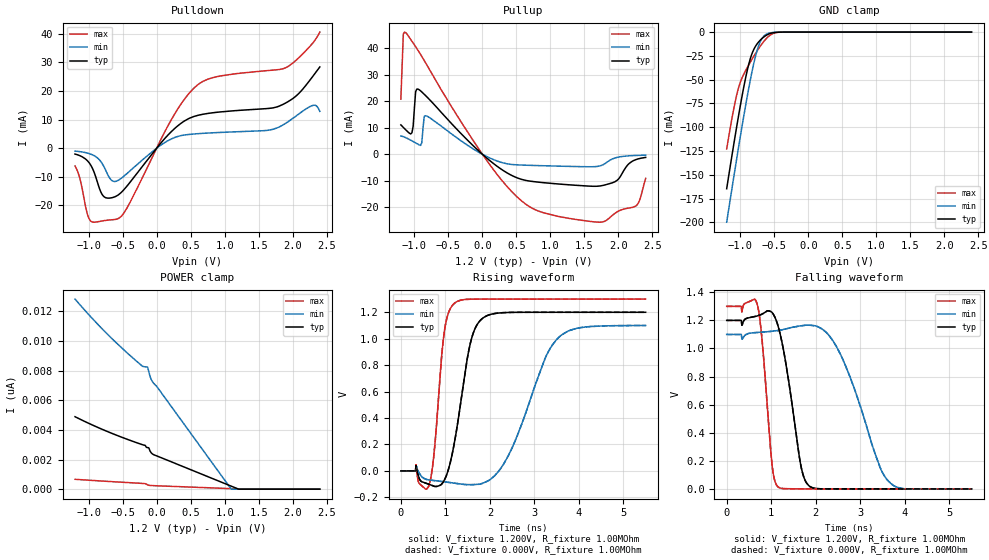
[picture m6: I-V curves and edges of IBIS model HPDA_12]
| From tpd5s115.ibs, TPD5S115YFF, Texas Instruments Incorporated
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[Model]   HPDA_12
Model_type   I/O
Vinl = 0.4V
Vinh = 1.0V
Vmeas = 1.500V
Vref = 0V
Cref =15pF
|   typ   min   max
|3-state
C_comp   1.5724pF   1.4611pF   1.8386pF
|pulldown
|C_comp   1.6216pF   1.4827pF   1.9515pF
|pullup
|C_comp   1.689pF   1.5267pF   2.0704pF
[Voltage Range]   1.200V   1.10V   1.30V
|Junction temperature
[Temperature Range]   40.0   100.0   -40.0
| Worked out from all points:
|   slope of the pulldown table from 0 to 0.18 V, typ, clamps not added: 36.5 ohm
|   slope of the pullup table from 0 to 0.18 V, typ, clamps not added: 47.1 ohm
|   GND clamp passes 1 mA (typ) near -0.54 V on its own axis
|   falling waveform, V_fixture 1.200V, R_fixture 1.00MOhm: 20-80 % time 333ps typ, 703ps min, 192ps max; typ from 1.2 V to 0 V
|   rising waveform, V_fixture 1.200V, R_fixture 1.00MOhm: 20-80 % time 340ps typ, 720ps min, 191ps max; typ from 0 V to 1.2 V
|   rising waveform, V_fixture 0.000V, R_fixture 1.00MOhm: 20-80 % time 340ps typ, 720ps min, 191ps max; typ from 0 V to 1.2 V
|   falling waveform, V_fixture 0.000V, R_fixture 1.00MOhm: 20-80 % time 333ps typ, 703ps min, 192ps max; typ from 1.2 V to 0 V
|ambient temperature   25   85   -40|
[Pulldown]
|   Voltage   I(typ)   I(min)   I(max)
-1.2V     -2.038mA   -994.7uA   -6.215mA
-982.9mV  -5.39mA    -1.945mA   -25.1mA
-783.9mV  -16.73mA   -6.042mA   -25.37mA
-675.4mV  -17.39mA   -10.91mA   -25.06mA
-566.8mV  -16.37mA   -11.25mA   -24.61mA
-385.9mV  -11.76mA   -7.802mA   -18.7mA
138.7mV   3.893mA    2.257mA    6.602mA
554.8mV   11.16mA    4.996mA    21.17mA
880.4mV   12.56mA    5.465mA    25mA
1.803V    14.74mA    7.446mA    27.54mA
2.291V    24.98mA    14.93mA    36.66mA
2.4V      28.44mA    12.91mA    40.63mA
[GND Clamp]
|   Voltage   I(typ)   I(min)   I(max)
-1.2V     -164.7mA   -199.9mA   -122.9mA
-1.11V    -124.1mA   -158.6mA   -85.69mA
-1.037V   -92.89mA   -126.4mA   -61.66mA
-982.9mV  -70.79mA   -102.8mA   -49.69mA
-874.4mV  -33.52mA   -58.6mA    -34.37mA
-820.1mV  -21.26mA   -39.03mA   -27.68mA
-747.7mV  -11.93mA   -18.1mA    -19.3mA
-693.5mV  -7.572mA   -8.233mA   -13.56mA
-639.2mV  -4.359mA   -3.305mA   -8.543mA
-530.7mV  -894.9uA   -472.7uA   -1.914mA
-404mV    -67.45uA   -43.38uA   -90.57uA
2.4V      0A         0A         0A
[Pullup]
|   Voltage   I(typ)   I(min)   I(max)
-1.2V     11.11mA    6.899mA    20.81mA
-1.164V   10.16mA    6.66mA     45.34mA
-1.146V   9.692mA    6.482mA    46.11mA
-1.037V   8.113mA    5.089mA    42.66mA
-982.9mV  23.63mA    4.314mA    40.6mA
-946.7mV  24.59mA    3.797mA    39.18mA
-892.5mV  23.54mA    4.317mA    36.94mA
-838.2mV  22.19mA    14.56mA    34.6mA
681.4mV   -10.04mA   -4.14mA    -19.58mA
1.767V    -11.76mA   -4.006mA   -25.49mA
2.273V    -1.845mA   -410.4uA   -19.07mA
2.4V      -1.169mA   -315.3uA   -9.052mA
[POWER Clamp]
|   Voltage   I(typ)   I(min)   I(max)
-1.2V     4.894nA    12.84nA    666.9pA
-874.4mV  4.189nA    11.18nA    569.1pA
-530.7mV  3.538nA    9.615nA    473.7pA
-205mV    2.998nA    8.296nA    384.9pA
-132.7mV  2.807nA    8.242nA    288.7pA
-114.6mV  2.792nA    7.924nA    264.5pA
-96.48mV  2.574nA    7.608nA    253.3pA
-60.3mV   2.374nA    7.251nA    242.1pA
0V        2.251nA    6.951nA    228.7pA
1.097V    202.6pA    0A         35.11pA
1.206V    0A         0A         15.96pA
2.4V      0A         0A         0A
[Ramp]
R_load = 1.00MOhm
|   typ   min   max
dV/dt_r   719.939mV/340.267ps 659.894mV/720.118ps 779.961mV/190.699ps
dV/dt_f   719.946mV/333.102ps 659.906mV/703.346ps 779.966mV/192.099ps
[Falling Waveform]
V_fixture = 1.200V
V_fixture_min = 1.100V
V_fixture_max = 1.300V
R_fixture = 1.00MOhm
|   Time   V(typ)   V(min)   V(max)
0s        1.2V       1.1V       1.3V
690ps     1.232V     1.114V     1.311V
800ps     1.246V     1.117V     1.043V
1.02ns    1.256V     1.123V     168.9mV
1.16ns    1.154V     1.128V     12.92mV
1.66ns    176.6mV    1.161V     538.2uV
1.85ns    21.76mV    1.166V     402.4uV
2.52ns    434.2uV    981.4mV    253.8uV
3.64ns    191.5uV    53.28mV    160.4uV
5.5ns     63.46uV    107.4uV    40.19uV
[Rising Waveform]
V_fixture = 1.200V
V_fixture_min = 1.100V
V_fixture_max = 1.300V
R_fixture = 1.00MOhm
|   Time   V(typ)   V(min)   V(max)
0s        63.46uV    107.4uV    40.19uV
630ps     -101.4mV   -68.14mV   -112.7mV
750ps     -116.4mV   -72.59mV   146.4mV
980ps     -67.29mV   -82.77mV   1.06V
1.22ns    246mV      -93.69mV   1.273V
1.56ns    964.1mV    -104.1mV   1.299V
1.86ns    1.16V      -90.66mV   1.3V
2.41ns    1.199V     113.1mV    1.3V
3.54ns    1.2V       1.008V     1.3V
5.5ns     1.2V       1.1V       1.3V
[Rising Waveform]
V_fixture = 0.000V
V_fixture_min = 0.000V
V_fixture_max = 0.000V
R_fixture = 1.00MOhm
|   Time   V(typ)   V(min)   V(max)
0s        23.36uV    46.82uV    14.13uV
630ps     -101.6mV   -68.32mV   -112.8mV
750ps     -116.6mV   -72.83mV   146.2mV
980ps     -67.63mV   -83.15mV   1.06V
1.22ns    245.6mV    -94.19mV   1.273V
1.56ns    963.9mV    -104.8mV   1.299V
1.86ns    1.16V      -91.45mV   1.3V
2.41ns    1.199V     112.2mV    1.3V
3.54ns    1.2V       1.008V     1.3V
5.5ns     1.2V       1.1V       1.3V
[Falling Waveform]
V_fixture = 0.000V
V_fixture_min = 0.000V
V_fixture_max = 0.000V
R_fixture = 1.00MOhm
|   Time   V(typ)   V(min)   V(max)
0s        1.2V       1.1V       1.3V
690ps     1.232V     1.114V     1.311V
800ps     1.246V     1.117V     1.043V
1.02ns    1.256V     1.123V     168.7mV
1.16ns    1.154V     1.128V     12.89mV
1.66ns    176.4mV    1.161V     511.9uV
1.85ns    21.69mV    1.166V     376.3uV
2.52ns    393.3uV    980.8mV    227.7uV
3.64ns    151.4uV    53.02mV    134.3uV
5.5ns     23.36uV    46.82uV    14.13uV
